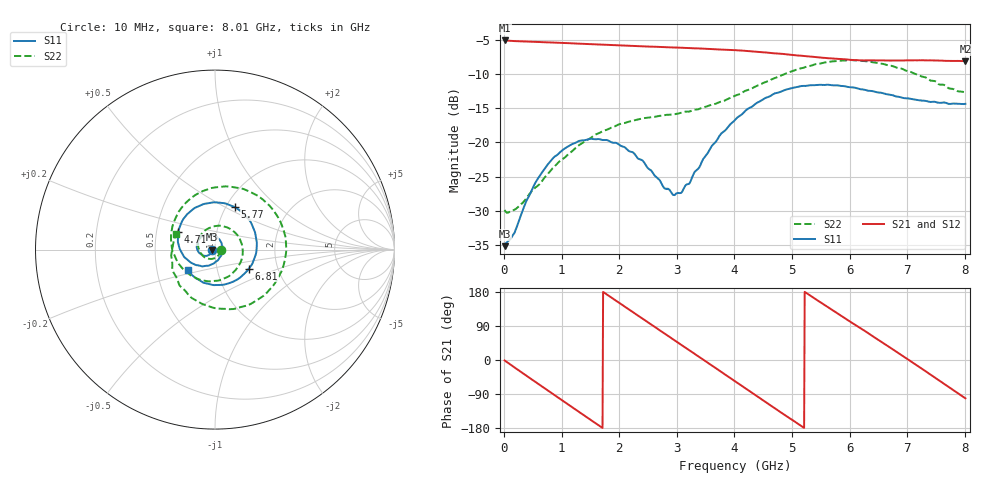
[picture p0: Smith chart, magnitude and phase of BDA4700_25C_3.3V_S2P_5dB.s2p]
!Agilent Technologies,E5071B,MY42404982,A.09.10
!Date: Mon Oct 20 18:05:05 2025
!Data & Calibration Information:
!Freq	S11:SOLT2(ON)	S21:SOLT2(ON)	S12:SOLT2(ON)	S22:SOLT2(ON)
# Hz S RI R 50
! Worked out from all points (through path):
!   801 points, 10 MHz to 8.01 GHz, reference 50 ohm
!   highest |S21| = -5.12 dB at 10 MHz (marker M1); lowest = -8.1 dB at 8.01 GHz (marker M2)
!   group delay of S21, straight-line fit = 284 ps
!   lowest |S11| = -35.2 dB at 10 MHz (marker M3), VSWR 1.04, Z = 48.3 - j0.11 ohm
!   |S11| at or under -10 dB: start of sweep to end of sweep
!   |S22| runs from -30.3 to -8.0 dB; largest |S21 - S12| = 0.0063
!   S11 on the Smith chart (normalised r, x): 10 MHz: 0.97, -0.00; 4.71 GHz: 0.65, +0.13; 5.77 GHz: 1.10, +0.56; 6.81 GHz: 1.42, -0.32; 8.01 GHz: 0.72, -0.17
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1e7  -0.0174 -0.00114  0.5546 -0.0118  0.554 -0.0123  0.032 -0.00263
3.3e8  -0.0241 -0.0216  0.4458 -0.3152  0.4455 -0.3154  0.0215 -0.0293
7.2e8  -0.0553 -0.0351  0.1278 -0.5227  0.1278 -0.5228  -0.0208 -0.0522
1.03e9  -0.0864 -0.0201  -0.1698 -0.5039  -0.1698 -0.5038  -0.0681 -0.0335
1.35e9  -0.102 0.0162  -0.4134 -0.3234  -0.4137 -0.3235  -0.0939 0.0283
1.64e9  -0.0906 0.0543  -0.5135 -0.0715  -0.5136 -0.0716  -0.069 0.0936
1.93e9  -0.0586 0.0802  -0.4746 0.1925  -0.4745 0.1926  0.00277 0.1312
2.32e9  -0.00385 0.0765  -0.2353 0.4458  -0.235 0.4459  0.1119 0.0948
2.68e9  0.0345 0.0415  0.0795 0.4915  0.0786 0.4909  0.1548 -0.015
2.97e9  0.0413 -0.00437  0.3091 0.3832  0.3088 0.3822  0.1197 -0.107
3.37e9  0.0106 -0.0632  0.4776 0.0842  0.4781 0.0838  -0.000678 -0.1742
3.67e9  -0.044 -0.0899  0.447 -0.1707  0.447 -0.1719  -0.1091 -0.1567
4.01e9  -0.1229 -0.0784  0.2629 -0.391  0.2634 -0.39  -0.2062 -0.0728
4.36e9  -0.1896 -0.00955  -0.0172 -0.4592  -0.0173 -0.4602  -0.2458 0.0689
4.71e9  -0.2062 0.0986  -0.2766 -0.3504  -0.2752 -0.3517  -0.1938 0.2233
5.35e9  -0.0508 0.2564  -0.4103 0.097  -0.411 0.095  0.118 0.345
5.77e9  0.1101 0.2364  -0.2335 0.3345  -0.2324 0.3346  0.3308 0.2118
6.19e9  0.2156 0.1149  0.043 0.3944  0.0482 0.3952  0.3915 -0.0452
6.68e9  0.2131 -0.0657  0.324 0.2269  0.3249 0.2264  0.2215 -0.2887
6.81e9  0.1882 -0.1063  0.3663 0.1488  0.3677 0.1461  0.1493 -0.3186
7.33e9  0.0382 -0.1967  0.3411 -0.2026  0.3412 -0.2036  -0.1391 -0.2616
8.01e9  -0.1526 -0.1151  -0.0759 -0.3841  -0.0746 -0.3844  -0.2165 0.0846
